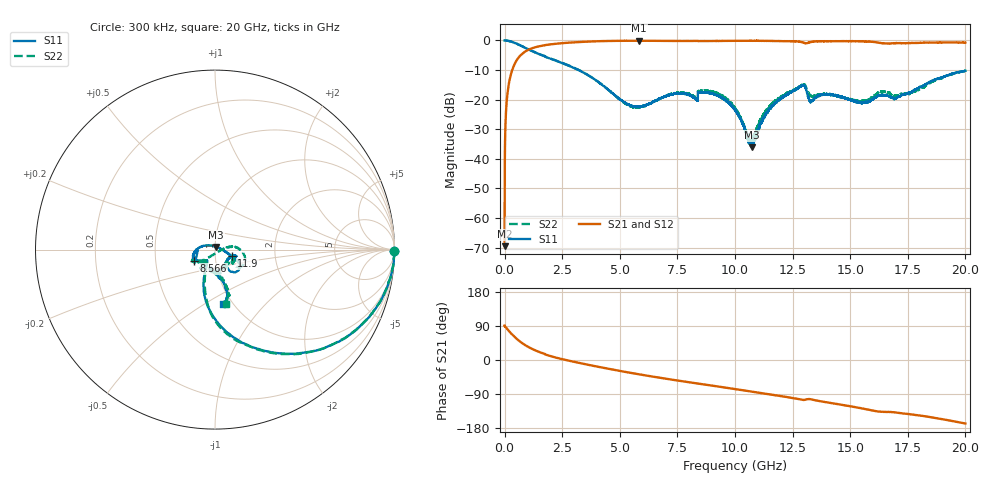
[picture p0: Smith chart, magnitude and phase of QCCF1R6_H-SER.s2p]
!{QCCF1R6}
!Johanson Technology Inc.
!www.johansontechnology.com
!Test Board Conditions:
!Substrate Type  RO4350B
!Substrate Thickness  10 mil
!Substrate Dk  3.66
!TL Type: GCPW
!TL Trace Width  21 mil
!TL Gap  20 mil
!Electrode orientation  Horizontal
!DUT TOPOLOGY	SERIES
!Mounting Pad LxW  16x21 mil
! Created Sat Jan  9 18:10:57 2021
# hz S ma R 50
! 2 Port Network Data from SP1.SP block
! freq  magS11  angS11  magS21  angS21  magS12  angS12  magS22  angS22
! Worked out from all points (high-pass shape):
!   20001 points, 300 kHz to 20 GHz, reference 50 ohm
!   highest |S21| = -0.09 dB at 5.842 GHz (marker M1); lowest = -69.5 dB at 300 kHz (marker M2)
!   |S21| within 3 dB of the highest: 1.046617 GHz to 1.048246 GHz (1.629 MHz wide, 0.155 % of centre); 1.048 GHz to end of sweep
!   lowest |S11| = -36.1 dB at 10.73 GHz (marker M3), VSWR 1.03, Z = 50.6 + j1.46 ohm
!   |S11| at or under -10 dB: 3.206 GHz to end of sweep
!   |S22| runs from -35.1 to 0.0 dB; largest |S21 - S12| = 0.014
!   S11 on the Smith chart (normalised r, x): 300 kHz: open; 8.566 GHz: 0.79, -0.10; 11.9 GHz: 1.20, -0.09; 20 GHz: 0.90, -0.60
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300000  0.9998 -0.4  0.0003342 90.7  0.0003941 93.8  0.9996 -0.5
1.013e8  0.993 -7.1  0.1033 82.6  0.1033 82.7  0.9937 -7.1
1.303e8  0.9901 -9.1  0.1323 80.6  0.1325 80.6  0.9907 -9.1
2.603e8  0.9634 -17.8  0.2563 71.5  0.2561 71.6  0.9638 -17.7
4.773e8  0.8969 -30.9  0.4306 58.5  0.4303 58.5  0.8967 -30.8
1.5353e9  0.5809 -69.2  0.8011 20.4  0.8039 20.4  0.5837 -69.1
3.3343e9  0.298 -99.4  0.9447 -8.9  0.9456 -9.0  0.3008 -98.2
5.8423e9  0.07516 -127.2  0.9892 -37.9  0.9869 -37.9  0.07362 -128.8
6.6673e9  0.1016 -141.6  0.9839 -46.2  0.9858 -46.2  0.101 -130.8
8.5663e9  0.1326 -151.7  0.9771 -63.9  0.9787 -63.8  0.1413 -153.7
9.3753e9  0.1102 -176.4  0.9802 -71.1  0.9809 -71.1  0.1197 -144.9
1.00003e10  0.06737 161.3  0.9856 -76.7  0.9857 -76.7  0.07236 -134.5
1.07283e10  0.01563 67.7  0.9856 -83.5  0.9848 -83.5  0.01846 -46.5
1.12903e10  0.05186 -9.3  0.9843 -88.6  0.9837 -88.7  0.05885 8.7
1.18993e10  0.09868 -21.3  0.9777 -94.5  0.9776 -94.4  0.106 9.0
1.29383e10  0.1736 -39.2  0.9275 -105.5  0.9276 -105.3  0.1799 -19.5
1.33343e10  0.09442 -31.4  0.9482 -104.0  0.9484 -104.1  0.114 -31.6
1.40373e10  0.1206 -17.1  0.9696 -112.3  0.9724 -112.2  0.1215 -32.7
1.54293e10  0.0901 -33.2  0.967 -126.8  0.9665 -126.9  0.0941 -50.2
1.66673e10  0.1153 -103.9  0.8858 -136.9  0.878 -137.3  0.1314 -99.2
1.76143e10  0.1327 -88.2  0.9027 -143.2  0.9033 -143.1  0.13 -88.9
2e10  0.3066 -81.5  0.92 -167.6  0.9118 -167.5  0.3078 -78.9
